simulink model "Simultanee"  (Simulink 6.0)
settings: Solver=ode45  StartTime=0  StopTime=3*t0  RelTol=1e-3
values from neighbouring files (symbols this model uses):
  beta = 0.95    [Constantes.m]    (also in ConstantesBck.m; ResCourV1.m = 1; ResCrV1.m = 1; ResEnerV1.m = 1)
  Cmem = 1E-6*Sm*(1-b)    (= 2.826e-08)    [Constantes.m]    (also in ConstantesBck.m = 3.14e-11; ImpedanceZtissus.m = 4e-08; Ztissus.m = 4e-08; CalculCharge.m = 1)
  N = [6,8,5,5,7,1,2,6,9,1,1,9,4,8,8,7]    [Constantes.m]    (also in ConstantesBck.m; ImpedanceZtissus.m = 100; Ztissus.m = 100; charge.m = N(:,2))
  rapportIE = 10    [Constantes.m]
  Rcan = 6.398E3*Sm*(1-b)    (= 180.80748)    [Constantes.m]    (also in ConstantesBck.m = 0.03454; ImpedanceZtissus.m = 44; Ztissus.m = 44)
  t0 = 2E-3    (= 0.002)    [Constantes.m]    (also in ConstantesBck.m = 0.001)
undefined symbols (not defined in the file or in its folder): ln
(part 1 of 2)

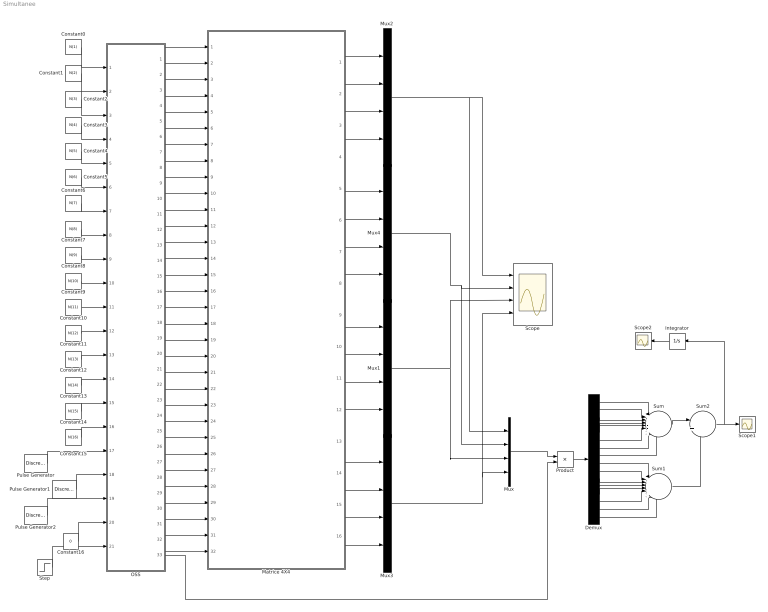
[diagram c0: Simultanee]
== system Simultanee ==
  Constant0 : Constant  Value=N(1)
  Constant1 : Constant  Value=N(2)
  Constant10 : Constant  Value=N(11)
  Constant11 : Constant  Value=N(12)
  Constant12 : Constant  Value=N(13)
  Constant13 : Constant  Value=N(14)
  Constant14 : Constant  Value=N(15)
  Constant15 : Constant  Value=N(16)
  Constant16 : Constant  Value=0
  Constant2 : Constant  Value=N(3)
  Constant3 : Constant  Value=N(4)
  Constant4 : Constant  Value=N(5)
  Constant5 : Constant  Value=N(6)
  Constant6 : Constant  Value=N(7)
  Constant7 : Constant  Value=N(8)
  Constant8 : Constant  Value=N(9)
  Constant9 : Constant  Value=N(10)
  Demux : Demux  Outputs=16
  Integrator : Integrator  Orientation=left
  Matrice 4X4 : Subsystem
  Mux{,1..4} (5 alike) : Mux
  OSS : Stateflow chart
  Product : Product
  Pulse Generator : DiscretePulseGenerator  PulseType=Time based  Period=2*t0  PulseWidth=50  PhaseDelay=2*t0
  Pulse Generator1 : DiscretePulseGenerator  PulseType=Time based  Period=4*t0  PulseWidth=50  PhaseDelay=3*t0
  Pulse Generator2 : DiscretePulseGenerator  PulseType=Time based  Period=8*t0  PulseWidth=50  PhaseDelay=5*t0
  Scope : Scope  NumInputPorts=4
  Scope1 : Scope
  Scope2 : Scope
  Step : Step  Time=t0  SampleTime=0
  Sum : Sum  Inputs=|++++++++
  Sum1 : Sum  Inputs=|++++++++
  Sum2 : Sum  Inputs=|++
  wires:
  Matrice 4X4/13(Out12) -> Mux3/1
  Matrice 4X4/14(Out13) -> Mux3/2
  Matrice 4X4/15(Out14) -> Mux3/3
  Matrice 4X4/16(Out15) -> Mux3/4
  Constant14/1 -> OSS/15(u14)
  Constant13/1 -> OSS/14(u13)
  Constant12/1 -> OSS/13(u12)
  Constant11/1 -> OSS/12(u11)
  Constant10/1 -> OSS/11(u10)
  Constant9/1 -> OSS/10(u9)
  Constant8/1 -> OSS/9(u8)
  Constant7/1 -> OSS/8(u7)
  Constant6/1 -> OSS/7(u6)
  Constant5/1 -> OSS/6(u5)
  Constant4/1 -> OSS/5(u4)
  Constant3/1 -> OSS/4(u3)
  Constant2/1 -> OSS/3(u2)
  Constant1/1 -> OSS/2(u1)
  Constant0/1 -> OSS/1(u0)
  Constant15/1 -> OSS/16(u15)
  OSS/5(S2) -> Matrice 4X4/5(S2)
  OSS/6(Ref2) -> Matrice 4X4/6(Ref2)
  OSS/7(S3) -> Matrice 4X4/7(S3)
  OSS/8(Ref3) -> Matrice 4X4/8(Ref3)
  OSS/9(S4) -> Matrice 4X4/9(S4)
  OSS/10(Ref4) -> Matrice 4X4/10(Ref4)
  OSS/11(S5) -> Matrice 4X4/11(S5)
  OSS/12(Ref5) -> Matrice 4X4/12(Ref5)
  OSS/13(S6) -> Matrice 4X4/13(S6)
  OSS/14(Ref6) -> Matrice 4X4/14(Ref6)
  OSS/15(S7) -> Matrice 4X4/15(S7)
  OSS/16(Ref7) -> Matrice 4X4/16(Ref7)
  OSS/17(S8) -> Matrice 4X4/17(S8)
  OSS/18(Ref8) -> Matrice 4X4/18(Ref8)
  OSS/19(S9) -> Matrice 4X4/19(S9)
  OSS/20(Ref9) -> Matrice 4X4/20(Ref9)
  OSS/21(S10) -> Matrice 4X4/21(S10)
  OSS/22(Ref10) -> Matrice 4X4/22(Ref10)
  OSS/23(S11) -> Matrice 4X4/23(S11)
  OSS/24(Ref11) -> Matrice 4X4/24(Ref11)
  OSS/25(S12) -> Matrice 4X4/25(S12)
  OSS/26(Ref12) -> Matrice 4X4/26(Ref12)
  OSS/27(S13) -> Matrice 4X4/27(S13)
  OSS/28(Ref13) -> Matrice 4X4/28(Ref13)
  OSS/29(S14) -> Matrice 4X4/29(S14)
  OSS/30(Ref14) -> Matrice 4X4/30(Ref14)
  OSS/31(S15) -> Matrice 4X4/31(S15)
  OSS/32(Ref15) -> Matrice 4X4/32(Ref15)
  OSS/4(Ref1) -> Matrice 4X4/4(Ref1)
  OSS/3(S1) -> Matrice 4X4/3(S1)
  OSS/2(Ref0) -> Matrice 4X4/2(Ref0)
  OSS/1(S0) -> Matrice 4X4/1(S0)
  Pulse Generator/1 -> OSS/17(tc0)
  Pulse Generator2/1 -> OSS/19(tc2)
  Pulse Generator1/1 -> OSS/18(tc1)
  Mux3/1 -> Mux/4, Scope/4
  Matrice 4X4/9(Out8) -> Mux1/1
  Matrice 4X4/10(Out9) -> Mux1/2
  Matrice 4X4/12(Out11) -> Mux1/4
  Matrice 4X4/11(Out10) -> Mux1/3
  Matrice 4X4/5(Out4) -> Mux4/1
  Matrice 4X4/6(Out5) -> Mux4/2
  Matrice 4X4/7(Out6) -> Mux4/3
  Matrice 4X4/8(Out7) -> Mux4/4
  Matrice 4X4/1(Out0) -> Mux2/1
  Matrice 4X4/2(Out1) -> Mux2/2
  Matrice 4X4/4(Out3) -> Mux2/4
  Matrice 4X4/3(Out2) -> Mux2/3
  Mux1/1 -> Mux/3, Scope/3
  Mux4/1 -> Mux/2, Scope/2
  Mux2/1 -> Mux/1, Scope/1
  Constant16/1 -> OSS/20(dyn)
  OSS/33(MatCourant) -> Product/2
  Mux/1 -> Product/1
  Product/1 -> Demux/1
  Demux/1 -> Sum/1
  Demux/2 -> Sum/2
  Demux/3 -> Sum/3
  Demux/4 -> Sum/4
  Demux/5 -> Sum/5
  Demux/6 -> Sum/6
  Demux/7 -> Sum/7
  Demux/8 -> Sum/8
  Demux/9 -> Sum1/1
  Demux/10 -> Sum1/2
  Demux/11 -> Sum1/3
  Demux/12 -> Sum1/4
  Demux/13 -> Sum1/5
  Demux/14 -> Sum1/6
  Demux/15 -> Sum1/7
  Demux/16 -> Sum1/8
  Sum/1 -> Sum2/1
  Sum1/1 -> Sum2/2
  Sum2/1 -> Scope1/1, Integrator/1
  Step/1 -> OSS/21(rst)
  Integrator/1 -> Scope2/1

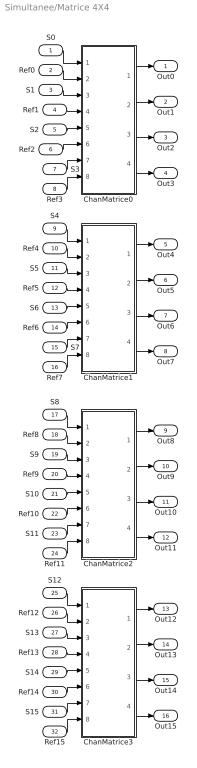
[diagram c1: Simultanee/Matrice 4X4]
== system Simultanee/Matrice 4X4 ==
  S0 : Inport  Port=1  LatchInput=off
  Ref0 : Inport  Port=2  LatchInput=off
  S1 : Inport  Port=3  LatchInput=off
  Ref1 : Inport  Port=4  LatchInput=off
  S2 : Inport  Port=5  LatchInput=off
  Ref2 : Inport  Port=6  LatchInput=off
  S3 : Inport  Port=7  LatchInput=off
  Ref3 : Inport  Port=8  LatchInput=off
  S4 : Inport  Port=9  LatchInput=off
  Ref4 : Inport  Port=10  LatchInput=off
  S5 : Inport  Port=11  LatchInput=off
  Ref5 : Inport  Port=12  LatchInput=off
  S6 : Inport  Port=13  LatchInput=off
  Ref6 : Inport  Port=14  LatchInput=off
  S7 : Inport  Port=15  LatchInput=off
  Ref7 : Inport  Port=16  LatchInput=off
  S8 : Inport  Port=17  LatchInput=off
  Ref8 : Inport  Port=18  LatchInput=off
  S9 : Inport  Port=19  LatchInput=off
  Ref9 : Inport  Port=20  LatchInput=off
  S10 : Inport  Port=21  LatchInput=off
  Ref10 : Inport  Port=22  LatchInput=off
  S11 : Inport  Port=23  LatchInput=off
  Ref11 : Inport  Port=24  LatchInput=off
  S12 : Inport  Port=25  LatchInput=off
  Ref12 : Inport  Port=26  LatchInput=off
  S13 : Inport  Port=27  LatchInput=off
  Ref13 : Inport  Port=28  LatchInput=off
  S14 : Inport  Port=29  LatchInput=off
  Ref14 : Inport  Port=30  LatchInput=off
  S15 : Inport  Port=31  LatchInput=off
  Ref15 : Inport  Port=32  LatchInput=off
  ChanMatrice0 : Subsystem
  ChanMatrice1 : Subsystem
  ChanMatrice2 : Subsystem
  ChanMatrice3 : Subsystem
  Out0 : Outport
  Out1 : Outport  Port=2
  Out2 : Outport  Port=3
  Out3 : Outport  Port=4
  Out4 : Outport  Port=5
  Out5 : Outport  Port=6
  Out6 : Outport  Port=7
  Out7 : Outport  Port=8
  Out8 : Outport  Port=9
  Out9 : Outport  Port=10
  Out10 : Outport  Port=11
  Out11 : Outport  Port=12
  Out12 : Outport  Port=13
  Out13 : Outport  Port=14
  Out14 : Outport  Port=15
  Out15 : Outport  Port=16
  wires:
  S0/1 -> ChanMatrice0/1(S0)
  ChanMatrice0/1(Out0) -> Out0/1
  Ref0/1 -> ChanMatrice0/2(Ref0)
  S1/1 -> ChanMatrice0/3(S1)
  ChanMatrice0/2(Out1) -> Out1/1
  ChanMatrice0/3(Out2) -> Out2/1
  ChanMatrice0/4(Out3) -> Out3/1
  ChanMatrice1/1(Out0) -> Out4/1
  ChanMatrice1/2(Out1) -> Out5/1
  ChanMatrice1/3(Out2) -> Out6/1
  ChanMatrice1/4(Out3) -> Out7/1
  ChanMatrice2/1(Out0) -> Out8/1
  ChanMatrice2/2(Out1) -> Out9/1
  ChanMatrice2/3(Out2) -> Out10/1
  ChanMatrice2/4(Out3) -> Out11/1
  ChanMatrice3/1(Out0) -> Out12/1
  ChanMatrice3/2(Out1) -> Out13/1
  ChanMatrice3/3(Out2) -> Out14/1
  ChanMatrice3/4(Out3) -> Out15/1
  S2/1 -> ChanMatrice0/5(S2)
  S3/1 -> ChanMatrice0/7(S3)
  S4/1 -> ChanMatrice1/1(S0)
  S5/1 -> ChanMatrice1/3(S1)
  S6/1 -> ChanMatrice1/5(S2)
  S7/1 -> ChanMatrice1/7(S3)
  S12/1 -> ChanMatrice3/1(S0)
  S13/1 -> ChanMatrice3/3(S1)
  S14/1 -> ChanMatrice3/5(S2)
  S15/1 -> ChanMatrice3/7(S3)
  S8/1 -> ChanMatrice2/1(S0)
  S9/1 -> ChanMatrice2/3(S1)
  S10/1 -> ChanMatrice2/5(S2)
  S11/1 -> ChanMatrice2/7(S3)
  Ref1/1 -> ChanMatrice0/4(Ref1)
  Ref2/1 -> ChanMatrice0/6(Ref2)
  Ref3/1 -> ChanMatrice0/8(Ref3)
  Ref4/1 -> ChanMatrice1/2(Ref0)
  Ref5/1 -> ChanMatrice1/4(Ref1)
  Ref6/1 -> ChanMatrice1/6(Ref2)
  Ref7/1 -> ChanMatrice1/8(Ref3)
  Ref8/1 -> ChanMatrice2/2(Ref0)
  Ref9/1 -> ChanMatrice2/4(Ref1)
  Ref10/1 -> ChanMatrice2/6(Ref2)
  Ref11/1 -> ChanMatrice2/8(Ref3)
  Ref12/1 -> ChanMatrice3/2(Ref0)
  Ref13/1 -> ChanMatrice3/4(Ref1)
  Ref14/1 -> ChanMatrice3/6(Ref2)
  Ref15/1 -> ChanMatrice3/8(Ref3)

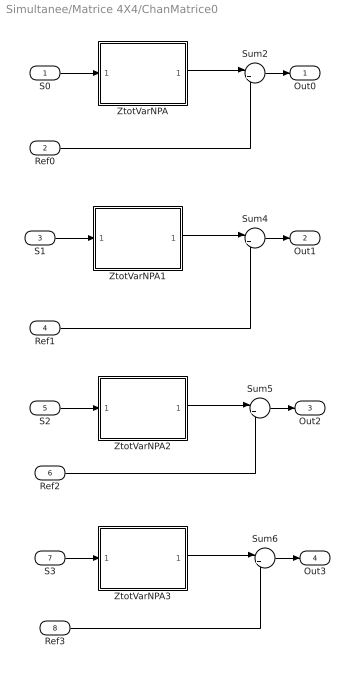
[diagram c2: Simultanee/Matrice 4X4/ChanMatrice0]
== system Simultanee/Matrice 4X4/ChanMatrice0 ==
  S0 : Inport  Port=1  LatchInput=off
  Ref0 : Inport  Port=2  LatchInput=off
  S1 : Inport  Port=3  LatchInput=off
  Ref1 : Inport  Port=4  LatchInput=off
  S2 : Inport  Port=5  LatchInput=off
  Ref2 : Inport  Port=6  LatchInput=off
  S3 : Inport  Port=7  LatchInput=off
  Ref3 : Inport  Port=8  LatchInput=off
  Sum{2,4..6} (4 alike) : Sum  Inputs=|++
  ZtotVarNPA : Subsystem
  ZtotVarNPA1 : Subsystem
  ZtotVarNPA2 : Subsystem
  ZtotVarNPA3 : Subsystem
  Out0 : Outport
  Out1 : Outport  Port=2
  Out2 : Outport  Port=3
  Out3 : Outport  Port=4
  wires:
  ZtotVarNPA/1(OutZtot) -> Sum2/1
  ZtotVarNPA1/1(OutZtot) -> Sum4/1
  ZtotVarNPA2/1(OutZtot) -> Sum5/1
  ZtotVarNPA3/1(OutZtot) -> Sum6/1
  Sum2/1 -> Out0/1
  S0/1 -> ZtotVarNPA/1(InZtot)
  Ref0/1 -> Sum2/2
  Sum4/1 -> Out1/1
  S1/1 -> ZtotVarNPA1/1(InZtot)
  Ref1/1 -> Sum4/2
  Sum5/1 -> Out2/1
  S2/1 -> ZtotVarNPA2/1(InZtot)
  Ref2/1 -> Sum5/2
  Sum6/1 -> Out3/1
  S3/1 -> ZtotVarNPA3/1(InZtot)
  Ref3/1 -> Sum6/2

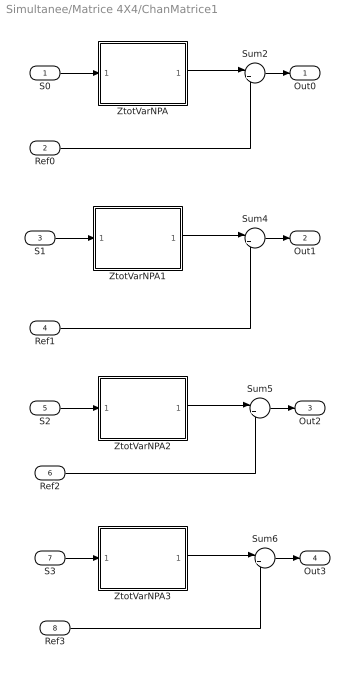
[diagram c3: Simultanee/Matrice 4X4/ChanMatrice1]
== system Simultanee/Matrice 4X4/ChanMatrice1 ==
  S0 : Inport  Port=1  LatchInput=off
  Ref0 : Inport  Port=2  LatchInput=off
  S1 : Inport  Port=3  LatchInput=off
  Ref1 : Inport  Port=4  LatchInput=off
  S2 : Inport  Port=5  LatchInput=off
  Ref2 : Inport  Port=6  LatchInput=off
  S3 : Inport  Port=7  LatchInput=off
  Ref3 : Inport  Port=8  LatchInput=off
  Sum{2,4..6} (4 alike) : Sum  Inputs=|++
  ZtotVarNPA : Subsystem
  ZtotVarNPA1 : Subsystem
  ZtotVarNPA2 : Subsystem
  ZtotVarNPA3 : Subsystem
  Out0 : Outport
  Out1 : Outport  Port=2
  Out2 : Outport  Port=3
  Out3 : Outport  Port=4
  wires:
  ZtotVarNPA/1(OutZtot) -> Sum2/1
  ZtotVarNPA1/1(OutZtot) -> Sum4/1
  ZtotVarNPA2/1(OutZtot) -> Sum5/1
  ZtotVarNPA3/1(OutZtot) -> Sum6/1
  Sum2/1 -> Out0/1
  S0/1 -> ZtotVarNPA/1(InZtot)
  Ref0/1 -> Sum2/2
  Sum4/1 -> Out1/1
  S1/1 -> ZtotVarNPA1/1(InZtot)
  Ref1/1 -> Sum4/2
  Sum5/1 -> Out2/1
  S2/1 -> ZtotVarNPA2/1(InZtot)
  Ref2/1 -> Sum5/2
  Sum6/1 -> Out3/1
  S3/1 -> ZtotVarNPA3/1(InZtot)
  Ref3/1 -> Sum6/2

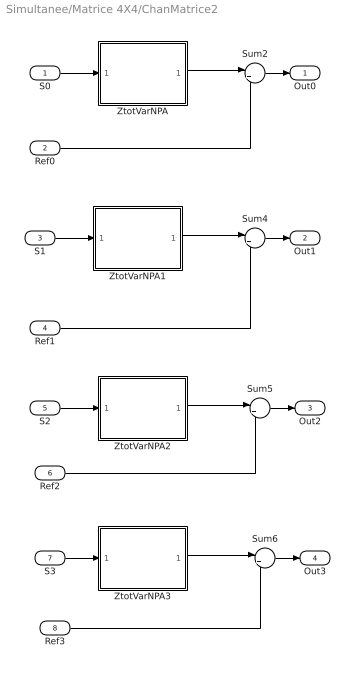
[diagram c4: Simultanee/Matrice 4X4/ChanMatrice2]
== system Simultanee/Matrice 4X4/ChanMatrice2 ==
  S0 : Inport  Port=1  LatchInput=off
  Ref0 : Inport  Port=2  LatchInput=off
  S1 : Inport  Port=3  LatchInput=off
  Ref1 : Inport  Port=4  LatchInput=off
  S2 : Inport  Port=5  LatchInput=off
  Ref2 : Inport  Port=6  LatchInput=off
  S3 : Inport  Port=7  LatchInput=off
  Ref3 : Inport  Port=8  LatchInput=off
  Sum{2,4..6} (4 alike) : Sum  Inputs=|++
  ZtotVarNPA : Subsystem
  ZtotVarNPA1 : Subsystem
  ZtotVarNPA2 : Subsystem
  ZtotVarNPA3 : Subsystem
  Out0 : Outport
  Out1 : Outport  Port=2
  Out2 : Outport  Port=3
  Out3 : Outport  Port=4
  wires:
  ZtotVarNPA/1(OutZtot) -> Sum2/1
  ZtotVarNPA1/1(OutZtot) -> Sum4/1
  ZtotVarNPA2/1(OutZtot) -> Sum5/1
  ZtotVarNPA3/1(OutZtot) -> Sum6/1
  Sum2/1 -> Out0/1
  S0/1 -> ZtotVarNPA/1(InZtot)
  Ref0/1 -> Sum2/2
  Sum4/1 -> Out1/1
  S1/1 -> ZtotVarNPA1/1(InZtot)
  Ref1/1 -> Sum4/2
  Sum5/1 -> Out2/1
  S2/1 -> ZtotVarNPA2/1(InZtot)
  Ref2/1 -> Sum5/2
  Sum6/1 -> Out3/1
  S3/1 -> ZtotVarNPA3/1(InZtot)
  Ref3/1 -> Sum6/2

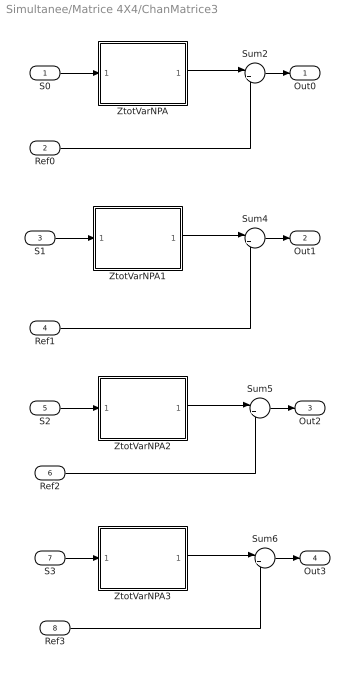
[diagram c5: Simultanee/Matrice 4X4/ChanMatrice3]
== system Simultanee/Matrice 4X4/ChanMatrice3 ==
  S0 : Inport  Port=1  LatchInput=off
  Ref0 : Inport  Port=2  LatchInput=off
  S1 : Inport  Port=3  LatchInput=off
  Ref1 : Inport  Port=4  LatchInput=off
  S2 : Inport  Port=5  LatchInput=off
  Ref2 : Inport  Port=6  LatchInput=off
  S3 : Inport  Port=7  LatchInput=off
  Ref3 : Inport  Port=8  LatchInput=off
  Sum{2,4..6} (4 alike) : Sum  Inputs=|++
  ZtotVarNPA : Subsystem
  ZtotVarNPA1 : Subsystem
  ZtotVarNPA2 : Subsystem
  ZtotVarNPA3 : Subsystem
  Out0 : Outport
  Out1 : Outport  Port=2
  Out2 : Outport  Port=3
  Out3 : Outport  Port=4
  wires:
  ZtotVarNPA/1(OutZtot) -> Sum2/1
  ZtotVarNPA1/1(OutZtot) -> Sum4/1
  ZtotVarNPA2/1(OutZtot) -> Sum5/1
  ZtotVarNPA3/1(OutZtot) -> Sum6/1
  Sum2/1 -> Out0/1
  S0/1 -> ZtotVarNPA/1(InZtot)
  Ref0/1 -> Sum2/2
  Sum4/1 -> Out1/1
  S1/1 -> ZtotVarNPA1/1(InZtot)
  Ref1/1 -> Sum4/2
  Sum5/1 -> Out2/1
  S2/1 -> ZtotVarNPA2/1(InZtot)
  Ref2/1 -> Sum5/2
  Sum6/1 -> Out3/1
  S3/1 -> ZtotVarNPA3/1(InZtot)
  Ref3/1 -> Sum6/2

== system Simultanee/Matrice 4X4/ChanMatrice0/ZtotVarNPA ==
  InZtot : Inport  Port=1  LatchInput=off
  Gain : Gain
  Sum : Sum  Inputs=|++
  ZietVar : Subsystem
  ZmembraneVar : Subsystem
  OutZtot : Outport
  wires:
  ZietVar/1(OutZiet) -> Gain/1
  ZmembraneVar/1(OutZmem) -> Sum/1
  InZtot/1 -> ZmembraneVar/1(InZmem), ZietVar/1(InZiet)
  Gain/1 -> Sum/2
  Sum/1 -> OutZtot/1

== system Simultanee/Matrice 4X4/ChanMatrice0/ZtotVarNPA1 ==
  InZtot : Inport  Port=1  LatchInput=off
  Gain : Gain
  Sum : Sum  Inputs=|++
  ZietVar : Subsystem
  ZmembraneVar : Subsystem
  OutZtot : Outport
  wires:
  ZietVar/1(OutZiet) -> Gain/1
  ZmembraneVar/1(OutZmem) -> Sum/1
  InZtot/1 -> ZmembraneVar/1(InZmem), ZietVar/1(InZiet)
  Gain/1 -> Sum/2
  Sum/1 -> OutZtot/1

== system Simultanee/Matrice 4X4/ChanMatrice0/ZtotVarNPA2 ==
  InZtot : Inport  Port=1  LatchInput=off
  Gain : Gain
  Sum : Sum  Inputs=|++
  ZietVar : Subsystem
  ZmembraneVar : Subsystem
  OutZtot : Outport
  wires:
  ZietVar/1(OutZiet) -> Gain/1
  ZmembraneVar/1(OutZmem) -> Sum/1
  InZtot/1 -> ZmembraneVar/1(InZmem), ZietVar/1(InZiet)
  Gain/1 -> Sum/2
  Sum/1 -> OutZtot/1

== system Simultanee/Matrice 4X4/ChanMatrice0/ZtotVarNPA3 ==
  InZtot : Inport  Port=1  LatchInput=off
  Gain : Gain
  Sum : Sum  Inputs=|++
  ZietVar : Subsystem
  ZmembraneVar : Subsystem
  OutZtot : Outport
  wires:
  ZietVar/1(OutZiet) -> Gain/1
  ZmembraneVar/1(OutZmem) -> Sum/1
  InZtot/1 -> ZmembraneVar/1(InZmem), ZietVar/1(InZiet)
  Gain/1 -> Sum/2
  Sum/1 -> OutZtot/1

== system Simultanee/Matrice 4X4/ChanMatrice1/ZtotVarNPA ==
  InZtot : Inport  Port=1  LatchInput=off
  Gain : Gain
  Sum : Sum  Inputs=|++
  ZietVar : Subsystem
  ZmembraneVar : Subsystem
  OutZtot : Outport
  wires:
  ZietVar/1(OutZiet) -> Gain/1
  ZmembraneVar/1(OutZmem) -> Sum/1
  InZtot/1 -> ZmembraneVar/1(InZmem), ZietVar/1(InZiet)
  Gain/1 -> Sum/2
  Sum/1 -> OutZtot/1

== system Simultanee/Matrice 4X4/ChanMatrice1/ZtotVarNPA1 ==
  InZtot : Inport  Port=1  LatchInput=off
  Gain : Gain
  Sum : Sum  Inputs=|++
  ZietVar : Subsystem
  ZmembraneVar : Subsystem
  OutZtot : Outport
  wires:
  ZietVar/1(OutZiet) -> Gain/1
  ZmembraneVar/1(OutZmem) -> Sum/1
  InZtot/1 -> ZmembraneVar/1(InZmem), ZietVar/1(InZiet)
  Gain/1 -> Sum/2
  Sum/1 -> OutZtot/1

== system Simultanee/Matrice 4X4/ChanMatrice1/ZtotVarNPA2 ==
  InZtot : Inport  Port=1  LatchInput=off
  Gain : Gain
  Sum : Sum  Inputs=|++
  ZietVar : Subsystem
  ZmembraneVar : Subsystem
  OutZtot : Outport
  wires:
  ZietVar/1(OutZiet) -> Gain/1
  ZmembraneVar/1(OutZmem) -> Sum/1
  InZtot/1 -> ZmembraneVar/1(InZmem), ZietVar/1(InZiet)
  Gain/1 -> Sum/2
  Sum/1 -> OutZtot/1

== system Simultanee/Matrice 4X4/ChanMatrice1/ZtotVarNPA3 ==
  InZtot : Inport  Port=1  LatchInput=off
  Gain : Gain
  Sum : Sum  Inputs=|++
  ZietVar : Subsystem
  ZmembraneVar : Subsystem
  OutZtot : Outport
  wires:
  ZietVar/1(OutZiet) -> Gain/1
  ZmembraneVar/1(OutZmem) -> Sum/1
  InZtot/1 -> ZmembraneVar/1(InZmem), ZietVar/1(InZiet)
  Gain/1 -> Sum/2
  Sum/1 -> OutZtot/1

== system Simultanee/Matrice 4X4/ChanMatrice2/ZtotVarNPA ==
  InZtot : Inport  Port=1  LatchInput=off
  Gain : Gain
  Sum : Sum  Inputs=|++
  ZietVar : Subsystem
  ZmembraneVar : Subsystem
  OutZtot : Outport
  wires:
  ZietVar/1(OutZiet) -> Gain/1
  ZmembraneVar/1(OutZmem) -> Sum/1
  InZtot/1 -> ZmembraneVar/1(InZmem), ZietVar/1(InZiet)
  Gain/1 -> Sum/2
  Sum/1 -> OutZtot/1

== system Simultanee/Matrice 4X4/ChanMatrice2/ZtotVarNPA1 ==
  InZtot : Inport  Port=1  LatchInput=off
  Gain : Gain
  Sum : Sum  Inputs=|++
  ZietVar : Subsystem
  ZmembraneVar : Subsystem
  OutZtot : Outport
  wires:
  ZietVar/1(OutZiet) -> Gain/1
  ZmembraneVar/1(OutZmem) -> Sum/1
  InZtot/1 -> ZmembraneVar/1(InZmem), ZietVar/1(InZiet)
  Gain/1 -> Sum/2
  Sum/1 -> OutZtot/1

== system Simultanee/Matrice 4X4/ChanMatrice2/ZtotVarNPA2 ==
  InZtot : Inport  Port=1  LatchInput=off
  Gain : Gain
  Sum : Sum  Inputs=|++
  ZietVar : Subsystem
  ZmembraneVar : Subsystem
  OutZtot : Outport
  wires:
  ZietVar/1(OutZiet) -> Gain/1
  ZmembraneVar/1(OutZmem) -> Sum/1
  InZtot/1 -> ZmembraneVar/1(InZmem), ZietVar/1(InZiet)
  Gain/1 -> Sum/2
  Sum/1 -> OutZtot/1

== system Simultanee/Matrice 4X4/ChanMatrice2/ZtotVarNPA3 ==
  InZtot : Inport  Port=1  LatchInput=off
  Gain : Gain
  Sum : Sum  Inputs=|++
  ZietVar : Subsystem
  ZmembraneVar : Subsystem
  OutZtot : Outport
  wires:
  ZietVar/1(OutZiet) -> Gain/1
  ZmembraneVar/1(OutZmem) -> Sum/1
  InZtot/1 -> ZmembraneVar/1(InZmem), ZietVar/1(InZiet)
  Gain/1 -> Sum/2
  Sum/1 -> OutZtot/1

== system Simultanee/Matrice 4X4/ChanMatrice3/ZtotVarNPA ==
  InZtot : Inport  Port=1  LatchInput=off
  Gain : Gain
  Sum : Sum  Inputs=|++
  ZietVar : Subsystem
  ZmembraneVar : Subsystem
  OutZtot : Outport
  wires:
  ZietVar/1(OutZiet) -> Gain/1
  ZmembraneVar/1(OutZmem) -> Sum/1
  InZtot/1 -> ZmembraneVar/1(InZmem), ZietVar/1(InZiet)
  Gain/1 -> Sum/2
  Sum/1 -> OutZtot/1

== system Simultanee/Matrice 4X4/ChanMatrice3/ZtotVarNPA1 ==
  InZtot : Inport  Port=1  LatchInput=off
  Gain : Gain
  Sum : Sum  Inputs=|++
  ZietVar : Subsystem
  ZmembraneVar : Subsystem
  OutZtot : Outport
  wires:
  ZietVar/1(OutZiet) -> Gain/1
  ZmembraneVar/1(OutZmem) -> Sum/1
  InZtot/1 -> ZmembraneVar/1(InZmem), ZietVar/1(InZiet)
  Gain/1 -> Sum/2
  Sum/1 -> OutZtot/1

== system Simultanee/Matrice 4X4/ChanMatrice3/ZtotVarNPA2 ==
  InZtot : Inport  Port=1  LatchInput=off
  Gain : Gain
  Sum : Sum  Inputs=|++
  ZietVar : Subsystem
  ZmembraneVar : Subsystem
  OutZtot : Outport
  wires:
  ZietVar/1(OutZiet) -> Gain/1
  ZmembraneVar/1(OutZmem) -> Sum/1
  InZtot/1 -> ZmembraneVar/1(InZmem), ZietVar/1(InZiet)
  Gain/1 -> Sum/2
  Sum/1 -> OutZtot/1

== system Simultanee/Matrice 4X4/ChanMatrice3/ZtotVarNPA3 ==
  InZtot : Inport  Port=1  LatchInput=off
  Gain : Gain
  Sum : Sum  Inputs=|++
  ZietVar : Subsystem
  ZmembraneVar : Subsystem
  OutZtot : Outport
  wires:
  ZietVar/1(OutZiet) -> Gain/1
  ZmembraneVar/1(OutZmem) -> Sum/1
  InZtot/1 -> ZmembraneVar/1(InZmem), ZietVar/1(InZiet)
  Gain/1 -> Sum/2
  Sum/1 -> OutZtot/1

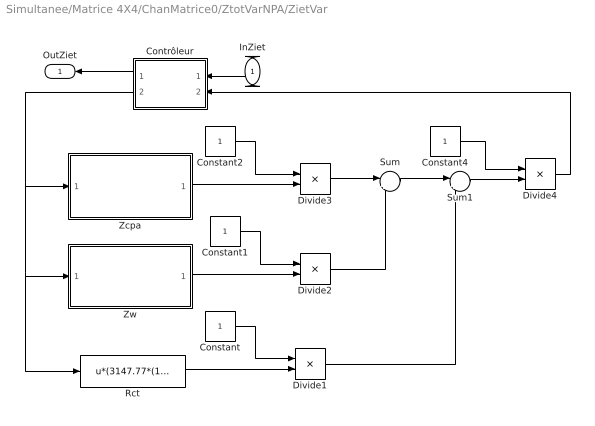
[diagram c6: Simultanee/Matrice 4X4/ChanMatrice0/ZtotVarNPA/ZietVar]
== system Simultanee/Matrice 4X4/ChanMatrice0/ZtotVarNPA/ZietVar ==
  InZiet : Inport  Orientation=left  Port=1  LatchInput=off
  Constant{,1..2,4} (4 alike) : Constant
  Contrôleur : Stateflow chart  Orientation=left
  Divide{1..4} (4 alike) : Product  Inputs=*/  OutScaling=2^-10
  Rct : Fcn  Expr=u*(3147.77*(1/((1E6*abs(u))^0.7199)))*1000
  Sum : Sum  Inputs=|++
  Sum1 : Sum  Inputs=|++
  Zcpa : Subsystem
  Zw : Subsystem
  OutZiet : Outport  Orientation=left
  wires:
  Constant/1 -> Divide1/1
  Constant1/1 -> Divide2/1
  Constant2/1 -> Divide3/1
  Zcpa/1(OutZcpa) -> Divide3/2
  Zw/1(OutZw) -> Divide2/2
  Rct/1 -> Divide1/2
  Divide3/1 -> Sum/1
  Constant4/1 -> Divide4/1
  Divide2/1 -> Sum/2
  Sum/1 -> Sum1/1
  Divide1/1 -> Sum1/2
  Sum1/1 -> Divide4/2
  Contrôleur/2(temp) -> Rct/1, Zw/1(InZw), Zcpa/1(InZcpa)
  InZiet/1 -> Contrôleur/1(u)
  Contrôleur/1(y) -> OutZiet/1
  Divide4/1 -> Contrôleur/2(calc)

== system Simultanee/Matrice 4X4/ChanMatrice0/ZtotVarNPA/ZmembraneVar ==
  InZmem : Inport  Orientation=left  Port=1  LatchInput=off
  Constant : Constant
  Constant1 : Constant
  Constant2 : Constant
  Contrôleur : Stateflow chart  Orientation=left
  Divide : Product  Inputs=*/  OutScaling=2^-10
  Divide1 : Product  Inputs=*/  OutScaling=2^-10
  Divide2 : Product  Inputs=*/  OutScaling=2^-10
  Gain : Gain  Gain=2
  Rext : Fcn  Expr=u*(1.6342*((abs(u)*1E6)^0.1267))*1E3
  Rint : Fcn  Expr=u*(1.6342*((abs(u)*1E6)^0.1267))*1E3/rapportIE
  Sum : Sum  Inputs=|++
  Sum1 : Sum  Inputs=|++
  Transfer Fcn : TransferFcn  Numerator=[Rcan]  Denominator=[Rcan*Cmem 1]
  OutZmem : Outport  Orientation=left
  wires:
  Gain/1 -> Transfer Fcn/1
  Transfer Fcn/1 -> Sum/1
  Sum/1 -> Divide/2
  Rext/1 -> Divide1/2
  Constant1/1 -> Divide/1
  Constant/1 -> Divide1/1
  Divide/1 -> Sum1/1
  Constant2/1 -> Divide2/1
  Sum1/1 -> Divide2/2
  Rint/1 -> Sum/2
  Divide1/1 -> Sum1/2
  Contrôleur/2(temp) -> Rext/1, Rint/1, Gain/1
  Divide2/1 -> Contrôleur/2(calc)
  InZmem/1 -> Contrôleur/1(u)
  Contrôleur/1(y) -> OutZmem/1

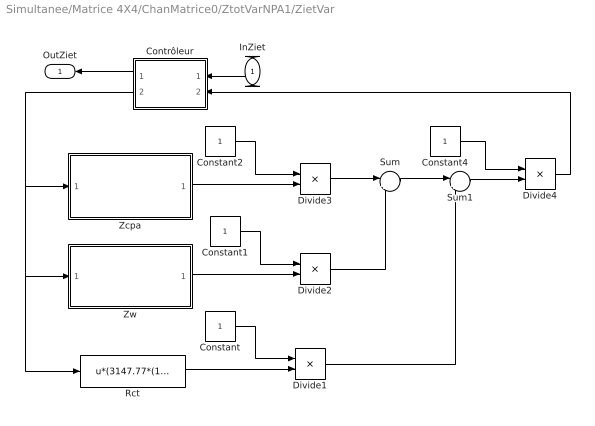
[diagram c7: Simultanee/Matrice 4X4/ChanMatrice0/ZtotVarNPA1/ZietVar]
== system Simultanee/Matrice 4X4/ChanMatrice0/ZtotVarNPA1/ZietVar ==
  InZiet : Inport  Orientation=left  Port=1  LatchInput=off
  Constant{,1..2,4} (4 alike) : Constant
  Contrôleur : Stateflow chart  Orientation=left
  Divide{1..4} (4 alike) : Product  Inputs=*/  OutScaling=2^-10
  Rct : Fcn  Expr=u*(3147.77*(1/((1E6*abs(u))^0.7199)))*1000
  Sum : Sum  Inputs=|++
  Sum1 : Sum  Inputs=|++
  Zcpa : Subsystem
  Zw : Subsystem
  OutZiet : Outport  Orientation=left
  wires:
  Constant/1 -> Divide1/1
  Constant1/1 -> Divide2/1
  Constant2/1 -> Divide3/1
  Zcpa/1(OutZcpa) -> Divide3/2
  Zw/1(OutZw) -> Divide2/2
  Rct/1 -> Divide1/2
  Divide3/1 -> Sum/1
  Constant4/1 -> Divide4/1
  Divide2/1 -> Sum/2
  Sum/1 -> Sum1/1
  Divide1/1 -> Sum1/2
  Sum1/1 -> Divide4/2
  Contrôleur/2(temp) -> Rct/1, Zw/1(InZw), Zcpa/1(InZcpa)
  InZiet/1 -> Contrôleur/1(u)
  Contrôleur/1(y) -> OutZiet/1
  Divide4/1 -> Contrôleur/2(calc)

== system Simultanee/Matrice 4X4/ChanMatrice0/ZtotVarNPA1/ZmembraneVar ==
  InZmem : Inport  Orientation=left  Port=1  LatchInput=off
  Constant : Constant
  Constant1 : Constant
  Constant2 : Constant
  Contrôleur : Stateflow chart  Orientation=left
  Divide : Product  Inputs=*/  OutScaling=2^-10
  Divide1 : Product  Inputs=*/  OutScaling=2^-10
  Divide2 : Product  Inputs=*/  OutScaling=2^-10
  Gain : Gain  Gain=2
  Rext : Fcn  Expr=u*(1.6342*((abs(u)*1E6)^0.1267))*1E3
  Rint : Fcn  Expr=u*(1.6342*((abs(u)*1E6)^0.1267))*1E3/rapportIE
  Sum : Sum  Inputs=|++
  Sum1 : Sum  Inputs=|++
  Transfer Fcn : TransferFcn  Numerator=[Rcan]  Denominator=[Rcan*Cmem 1]
  OutZmem : Outport  Orientation=left
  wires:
  Gain/1 -> Transfer Fcn/1
  Transfer Fcn/1 -> Sum/1
  Sum/1 -> Divide/2
  Rext/1 -> Divide1/2
  Constant1/1 -> Divide/1
  Constant/1 -> Divide1/1
  Divide/1 -> Sum1/1
  Constant2/1 -> Divide2/1
  Sum1/1 -> Divide2/2
  Rint/1 -> Sum/2
  Divide1/1 -> Sum1/2
  Contrôleur/2(temp) -> Rext/1, Rint/1, Gain/1
  Divide2/1 -> Contrôleur/2(calc)
  InZmem/1 -> Contrôleur/1(u)
  Contrôleur/1(y) -> OutZmem/1

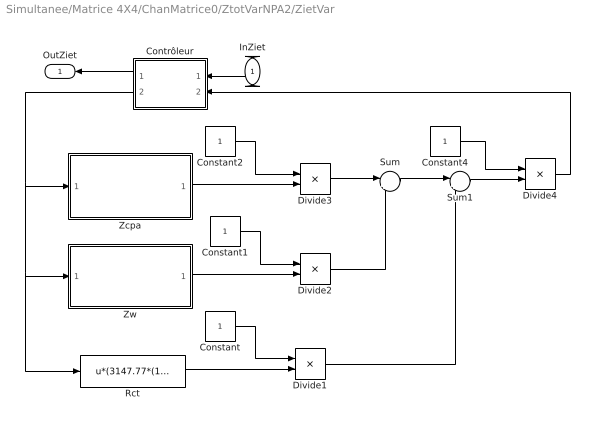
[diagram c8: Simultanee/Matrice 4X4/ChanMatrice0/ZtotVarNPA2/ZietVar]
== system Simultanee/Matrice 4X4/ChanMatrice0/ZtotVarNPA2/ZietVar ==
  InZiet : Inport  Orientation=left  Port=1  LatchInput=off
  Constant{,1..2,4} (4 alike) : Constant
  Contrôleur : Stateflow chart  Orientation=left
  Divide{1..4} (4 alike) : Product  Inputs=*/  OutScaling=2^-10
  Rct : Fcn  Expr=u*(3147.77*(1/((1E6*abs(u))^0.7199)))*1000
  Sum : Sum  Inputs=|++
  Sum1 : Sum  Inputs=|++
  Zcpa : Subsystem
  Zw : Subsystem
  OutZiet : Outport  Orientation=left
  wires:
  Constant/1 -> Divide1/1
  Constant1/1 -> Divide2/1
  Constant2/1 -> Divide3/1
  Zcpa/1(OutZcpa) -> Divide3/2
  Zw/1(OutZw) -> Divide2/2
  Rct/1 -> Divide1/2
  Divide3/1 -> Sum/1
  Constant4/1 -> Divide4/1
  Divide2/1 -> Sum/2
  Sum/1 -> Sum1/1
  Divide1/1 -> Sum1/2
  Sum1/1 -> Divide4/2
  Contrôleur/2(temp) -> Rct/1, Zw/1(InZw), Zcpa/1(InZcpa)
  InZiet/1 -> Contrôleur/1(u)
  Contrôleur/1(y) -> OutZiet/1
  Divide4/1 -> Contrôleur/2(calc)

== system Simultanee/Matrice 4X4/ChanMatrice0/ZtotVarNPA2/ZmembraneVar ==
  InZmem : Inport  Orientation=left  Port=1  LatchInput=off
  Constant : Constant
  Constant1 : Constant
  Constant2 : Constant
  Contrôleur : Stateflow chart  Orientation=left
  Divide : Product  Inputs=*/  OutScaling=2^-10
  Divide1 : Product  Inputs=*/  OutScaling=2^-10
  Divide2 : Product  Inputs=*/  OutScaling=2^-10
  Gain : Gain  Gain=2
  Rext : Fcn  Expr=u*(1.6342*((abs(u)*1E6)^0.1267))*1E3
  Rint : Fcn  Expr=u*(1.6342*((abs(u)*1E6)^0.1267))*1E3/rapportIE
  Sum : Sum  Inputs=|++
  Sum1 : Sum  Inputs=|++
  Transfer Fcn : TransferFcn  Numerator=[Rcan]  Denominator=[Rcan*Cmem 1]
  OutZmem : Outport  Orientation=left
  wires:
  Gain/1 -> Transfer Fcn/1
  Transfer Fcn/1 -> Sum/1
  Sum/1 -> Divide/2
  Rext/1 -> Divide1/2
  Constant1/1 -> Divide/1
  Constant/1 -> Divide1/1
  Divide/1 -> Sum1/1
  Constant2/1 -> Divide2/1
  Sum1/1 -> Divide2/2
  Rint/1 -> Sum/2
  Divide1/1 -> Sum1/2
  Contrôleur/2(temp) -> Rext/1, Rint/1, Gain/1
  Divide2/1 -> Contrôleur/2(calc)
  InZmem/1 -> Contrôleur/1(u)
  Contrôleur/1(y) -> OutZmem/1

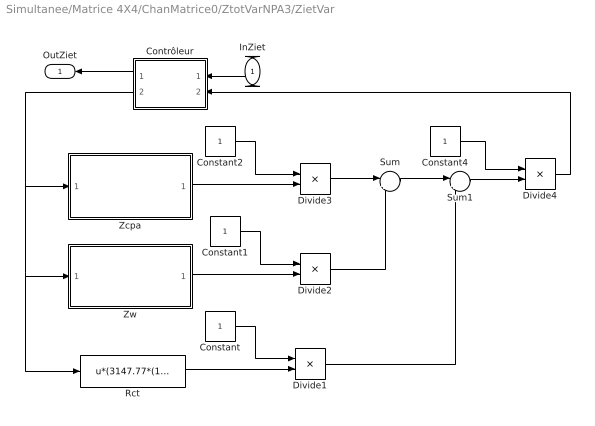
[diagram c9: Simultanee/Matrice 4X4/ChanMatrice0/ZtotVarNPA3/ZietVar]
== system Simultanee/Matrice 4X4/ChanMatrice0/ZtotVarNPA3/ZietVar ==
  InZiet : Inport  Orientation=left  Port=1  LatchInput=off
  Constant{,1..2,4} (4 alike) : Constant
  Contrôleur : Stateflow chart  Orientation=left
  Divide{1..4} (4 alike) : Product  Inputs=*/  OutScaling=2^-10
  Rct : Fcn  Expr=u*(3147.77*(1/((1E6*abs(u))^0.7199)))*1000
  Sum : Sum  Inputs=|++
  Sum1 : Sum  Inputs=|++
  Zcpa : Subsystem
  Zw : Subsystem
  OutZiet : Outport  Orientation=left
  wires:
  Constant/1 -> Divide1/1
  Constant1/1 -> Divide2/1
  Constant2/1 -> Divide3/1
  Zcpa/1(OutZcpa) -> Divide3/2
  Zw/1(OutZw) -> Divide2/2
  Rct/1 -> Divide1/2
  Divide3/1 -> Sum/1
  Constant4/1 -> Divide4/1
  Divide2/1 -> Sum/2
  Sum/1 -> Sum1/1
  Divide1/1 -> Sum1/2
  Sum1/1 -> Divide4/2
  Contrôleur/2(temp) -> Rct/1, Zw/1(InZw), Zcpa/1(InZcpa)
  InZiet/1 -> Contrôleur/1(u)
  Contrôleur/1(y) -> OutZiet/1
  Divide4/1 -> Contrôleur/2(calc)

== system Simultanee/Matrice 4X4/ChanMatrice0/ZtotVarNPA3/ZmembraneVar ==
  InZmem : Inport  Orientation=left  Port=1  LatchInput=off
  Constant : Constant
  Constant1 : Constant
  Constant2 : Constant
  Contrôleur : Stateflow chart  Orientation=left
  Divide : Product  Inputs=*/  OutScaling=2^-10
  Divide1 : Product  Inputs=*/  OutScaling=2^-10
  Divide2 : Product  Inputs=*/  OutScaling=2^-10
  Gain : Gain  Gain=2
  Rext : Fcn  Expr=u*(1.6342*((abs(u)*1E6)^0.1267))*1E3
  Rint : Fcn  Expr=u*(1.6342*((abs(u)*1E6)^0.1267))*1E3/rapportIE
  Sum : Sum  Inputs=|++
  Sum1 : Sum  Inputs=|++
  Transfer Fcn : TransferFcn  Numerator=[Rcan]  Denominator=[Rcan*Cmem 1]
  OutZmem : Outport  Orientation=left
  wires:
  Gain/1 -> Transfer Fcn/1
  Transfer Fcn/1 -> Sum/1
  Sum/1 -> Divide/2
  Rext/1 -> Divide1/2
  Constant1/1 -> Divide/1
  Constant/1 -> Divide1/1
  Divide/1 -> Sum1/1
  Constant2/1 -> Divide2/1
  Sum1/1 -> Divide2/2
  Rint/1 -> Sum/2
  Divide1/1 -> Sum1/2
  Contrôleur/2(temp) -> Rext/1, Rint/1, Gain/1
  Divide2/1 -> Contrôleur/2(calc)
  InZmem/1 -> Contrôleur/1(u)
  Contrôleur/1(y) -> OutZmem/1

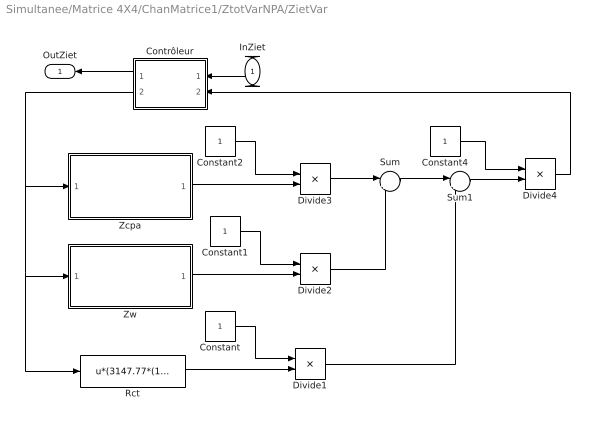
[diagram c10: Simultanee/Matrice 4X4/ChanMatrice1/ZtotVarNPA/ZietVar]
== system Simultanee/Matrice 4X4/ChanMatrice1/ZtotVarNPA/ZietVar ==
  InZiet : Inport  Orientation=left  Port=1  LatchInput=off
  Constant{,1..2,4} (4 alike) : Constant
  Contrôleur : Stateflow chart  Orientation=left
  Divide{1..4} (4 alike) : Product  Inputs=*/  OutScaling=2^-10
  Rct : Fcn  Expr=u*(3147.77*(1/((1E6*abs(u))^0.7199)))*1000
  Sum : Sum  Inputs=|++
  Sum1 : Sum  Inputs=|++
  Zcpa : Subsystem
  Zw : Subsystem
  OutZiet : Outport  Orientation=left
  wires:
  Constant/1 -> Divide1/1
  Constant1/1 -> Divide2/1
  Constant2/1 -> Divide3/1
  Zcpa/1(OutZcpa) -> Divide3/2
  Zw/1(OutZw) -> Divide2/2
  Rct/1 -> Divide1/2
  Divide3/1 -> Sum/1
  Constant4/1 -> Divide4/1
  Divide2/1 -> Sum/2
  Sum/1 -> Sum1/1
  Divide1/1 -> Sum1/2
  Sum1/1 -> Divide4/2
  Contrôleur/2(temp) -> Rct/1, Zw/1(InZw), Zcpa/1(InZcpa)
  InZiet/1 -> Contrôleur/1(u)
  Contrôleur/1(y) -> OutZiet/1
  Divide4/1 -> Contrôleur/2(calc)

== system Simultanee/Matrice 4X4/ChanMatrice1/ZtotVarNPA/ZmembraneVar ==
  InZmem : Inport  Orientation=left  Port=1  LatchInput=off
  Constant : Constant
  Constant1 : Constant
  Constant2 : Constant
  Contrôleur : Stateflow chart  Orientation=left
  Divide : Product  Inputs=*/  OutScaling=2^-10
  Divide1 : Product  Inputs=*/  OutScaling=2^-10
  Divide2 : Product  Inputs=*/  OutScaling=2^-10
  Gain : Gain  Gain=2
  Rext : Fcn  Expr=u*(1.6342*((abs(u)*1E6)^0.1267))*1E3
  Rint : Fcn  Expr=u*(1.6342*((abs(u)*1E6)^0.1267))*1E3/rapportIE
  Sum : Sum  Inputs=|++
  Sum1 : Sum  Inputs=|++
  Transfer Fcn : TransferFcn  Numerator=[Rcan]  Denominator=[Rcan*Cmem 1]
  OutZmem : Outport  Orientation=left
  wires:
  Gain/1 -> Transfer Fcn/1
  Transfer Fcn/1 -> Sum/1
  Sum/1 -> Divide/2
  Rext/1 -> Divide1/2
  Constant1/1 -> Divide/1
  Constant/1 -> Divide1/1
  Divide/1 -> Sum1/1
  Constant2/1 -> Divide2/1
  Sum1/1 -> Divide2/2
  Rint/1 -> Sum/2
  Divide1/1 -> Sum1/2
  Contrôleur/2(temp) -> Rext/1, Rint/1, Gain/1
  Divide2/1 -> Contrôleur/2(calc)
  InZmem/1 -> Contrôleur/1(u)
  Contrôleur/1(y) -> OutZmem/1

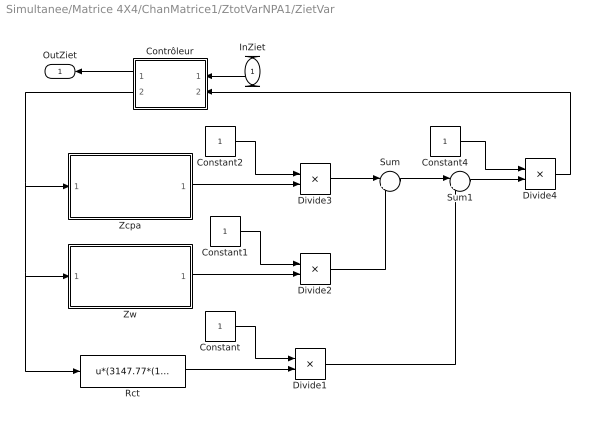
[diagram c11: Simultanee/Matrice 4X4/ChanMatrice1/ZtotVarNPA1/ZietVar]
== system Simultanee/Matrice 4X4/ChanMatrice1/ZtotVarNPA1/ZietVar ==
  InZiet : Inport  Orientation=left  Port=1  LatchInput=off
  Constant{,1..2,4} (4 alike) : Constant
  Contrôleur : Stateflow chart  Orientation=left
  Divide{1..4} (4 alike) : Product  Inputs=*/  OutScaling=2^-10
  Rct : Fcn  Expr=u*(3147.77*(1/((1E6*abs(u))^0.7199)))*1000
  Sum : Sum  Inputs=|++
  Sum1 : Sum  Inputs=|++
  Zcpa : Subsystem
  Zw : Subsystem
  OutZiet : Outport  Orientation=left
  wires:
  Constant/1 -> Divide1/1
  Constant1/1 -> Divide2/1
  Constant2/1 -> Divide3/1
  Zcpa/1(OutZcpa) -> Divide3/2
  Zw/1(OutZw) -> Divide2/2
  Rct/1 -> Divide1/2
  Divide3/1 -> Sum/1
  Constant4/1 -> Divide4/1
  Divide2/1 -> Sum/2
  Sum/1 -> Sum1/1
  Divide1/1 -> Sum1/2
  Sum1/1 -> Divide4/2
  Contrôleur/2(temp) -> Rct/1, Zw/1(InZw), Zcpa/1(InZcpa)
  InZiet/1 -> Contrôleur/1(u)
  Contrôleur/1(y) -> OutZiet/1
  Divide4/1 -> Contrôleur/2(calc)

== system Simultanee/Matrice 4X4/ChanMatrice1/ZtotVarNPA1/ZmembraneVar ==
  InZmem : Inport  Orientation=left  Port=1  LatchInput=off
  Constant : Constant
  Constant1 : Constant
  Constant2 : Constant
  Contrôleur : Stateflow chart  Orientation=left
  Divide : Product  Inputs=*/  OutScaling=2^-10
  Divide1 : Product  Inputs=*/  OutScaling=2^-10
  Divide2 : Product  Inputs=*/  OutScaling=2^-10
  Gain : Gain  Gain=2
  Rext : Fcn  Expr=u*(1.6342*((abs(u)*1E6)^0.1267))*1E3
  Rint : Fcn  Expr=u*(1.6342*((abs(u)*1E6)^0.1267))*1E3/rapportIE
  Sum : Sum  Inputs=|++
  Sum1 : Sum  Inputs=|++
  Transfer Fcn : TransferFcn  Numerator=[Rcan]  Denominator=[Rcan*Cmem 1]
  OutZmem : Outport  Orientation=left
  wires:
  Gain/1 -> Transfer Fcn/1
  Transfer Fcn/1 -> Sum/1
  Sum/1 -> Divide/2
  Rext/1 -> Divide1/2
  Constant1/1 -> Divide/1
  Constant/1 -> Divide1/1
  Divide/1 -> Sum1/1
  Constant2/1 -> Divide2/1
  Sum1/1 -> Divide2/2
  Rint/1 -> Sum/2
  Divide1/1 -> Sum1/2
  Contrôleur/2(temp) -> Rext/1, Rint/1, Gain/1
  Divide2/1 -> Contrôleur/2(calc)
  InZmem/1 -> Contrôleur/1(u)
  Contrôleur/1(y) -> OutZmem/1

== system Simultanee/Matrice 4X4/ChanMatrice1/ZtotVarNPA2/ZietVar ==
  InZiet : Inport  Orientation=left  Port=1  LatchInput=off
  Constant{,1..2,4} (4 alike) : Constant
  Contrôleur : Stateflow chart  Orientation=left
  Divide{1..4} (4 alike) : Product  Inputs=*/  OutScaling=2^-10
  Rct : Fcn  Expr=u*(3147.77*(1/((1E6*abs(u))^0.7199)))*1000
  Sum : Sum  Inputs=|++
  Sum1 : Sum  Inputs=|++
  Zcpa : Subsystem
  Zw : Subsystem
  OutZiet : Outport  Orientation=left
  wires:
  Constant/1 -> Divide1/1
  Constant1/1 -> Divide2/1
  Constant2/1 -> Divide3/1
  Zcpa/1(OutZcpa) -> Divide3/2
  Zw/1(OutZw) -> Divide2/2
  Rct/1 -> Divide1/2
  Divide3/1 -> Sum/1
  Constant4/1 -> Divide4/1
  Divide2/1 -> Sum/2
  Sum/1 -> Sum1/1
  Divide1/1 -> Sum1/2
  Sum1/1 -> Divide4/2
  Contrôleur/2(temp) -> Rct/1, Zw/1(InZw), Zcpa/1(InZcpa)
  InZiet/1 -> Contrôleur/1(u)
  Contrôleur/1(y) -> OutZiet/1
  Divide4/1 -> Contrôleur/2(calc)

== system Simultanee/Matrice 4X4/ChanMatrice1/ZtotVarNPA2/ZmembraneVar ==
  InZmem : Inport  Orientation=left  Port=1  LatchInput=off
  Constant : Constant
  Constant1 : Constant
  Constant2 : Constant
  Contrôleur : Stateflow chart  Orientation=left
  Divide : Product  Inputs=*/  OutScaling=2^-10
  Divide1 : Product  Inputs=*/  OutScaling=2^-10
  Divide2 : Product  Inputs=*/  OutScaling=2^-10
  Gain : Gain  Gain=2
  Rext : Fcn  Expr=u*(1.6342*((abs(u)*1E6)^0.1267))*1E3
  Rint : Fcn  Expr=u*(1.6342*((abs(u)*1E6)^0.1267))*1E3/rapportIE
  Sum : Sum  Inputs=|++
  Sum1 : Sum  Inputs=|++
  Transfer Fcn : TransferFcn  Numerator=[Rcan]  Denominator=[Rcan*Cmem 1]
  OutZmem : Outport  Orientation=left
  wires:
  Gain/1 -> Transfer Fcn/1
  Transfer Fcn/1 -> Sum/1
  Sum/1 -> Divide/2
  Rext/1 -> Divide1/2
  Constant1/1 -> Divide/1
  Constant/1 -> Divide1/1
  Divide/1 -> Sum1/1
  Constant2/1 -> Divide2/1
  Sum1/1 -> Divide2/2
  Rint/1 -> Sum/2
  Divide1/1 -> Sum1/2
  Contrôleur/2(temp) -> Rext/1, Rint/1, Gain/1
  Divide2/1 -> Contrôleur/2(calc)
  InZmem/1 -> Contrôleur/1(u)
  Contrôleur/1(y) -> OutZmem/1

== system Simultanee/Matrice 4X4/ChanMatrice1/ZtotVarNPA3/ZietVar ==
  InZiet : Inport  Orientation=left  Port=1  LatchInput=off
  Constant{,1..2,4} (4 alike) : Constant
  Contrôleur : Stateflow chart  Orientation=left
  Divide{1..4} (4 alike) : Product  Inputs=*/  OutScaling=2^-10
  Rct : Fcn  Expr=u*(3147.77*(1/((1E6*abs(u))^0.7199)))*1000
  Sum : Sum  Inputs=|++
  Sum1 : Sum  Inputs=|++
  Zcpa : Subsystem
  Zw : Subsystem
  OutZiet : Outport  Orientation=left
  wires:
  Constant/1 -> Divide1/1
  Constant1/1 -> Divide2/1
  Constant2/1 -> Divide3/1
  Zcpa/1(OutZcpa) -> Divide3/2
  Zw/1(OutZw) -> Divide2/2
  Rct/1 -> Divide1/2
  Divide3/1 -> Sum/1
  Constant4/1 -> Divide4/1
  Divide2/1 -> Sum/2
  Sum/1 -> Sum1/1
  Divide1/1 -> Sum1/2
  Sum1/1 -> Divide4/2
  Contrôleur/2(temp) -> Rct/1, Zw/1(InZw), Zcpa/1(InZcpa)
  InZiet/1 -> Contrôleur/1(u)
  Contrôleur/1(y) -> OutZiet/1
  Divide4/1 -> Contrôleur/2(calc)

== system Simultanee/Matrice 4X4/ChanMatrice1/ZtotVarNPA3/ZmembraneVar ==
  InZmem : Inport  Orientation=left  Port=1  LatchInput=off
  Constant : Constant
  Constant1 : Constant
  Constant2 : Constant
  Contrôleur : Stateflow chart  Orientation=left
  Divide : Product  Inputs=*/  OutScaling=2^-10
  Divide1 : Product  Inputs=*/  OutScaling=2^-10
  Divide2 : Product  Inputs=*/  OutScaling=2^-10
  Gain : Gain  Gain=2
  Rext : Fcn  Expr=u*(1.6342*((abs(u)*1E6)^0.1267))*1E3
  Rint : Fcn  Expr=u*(1.6342*((abs(u)*1E6)^0.1267))*1E3/rapportIE
  Sum : Sum  Inputs=|++
  Sum1 : Sum  Inputs=|++
  Transfer Fcn : TransferFcn  Numerator=[Rcan]  Denominator=[Rcan*Cmem 1]
  OutZmem : Outport  Orientation=left
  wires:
  Gain/1 -> Transfer Fcn/1
  Transfer Fcn/1 -> Sum/1
  Sum/1 -> Divide/2
  Rext/1 -> Divide1/2
  Constant1/1 -> Divide/1
  Constant/1 -> Divide1/1
  Divide/1 -> Sum1/1
  Constant2/1 -> Divide2/1
  Sum1/1 -> Divide2/2
  Rint/1 -> Sum/2
  Divide1/1 -> Sum1/2
  Contrôleur/2(temp) -> Rext/1, Rint/1, Gain/1
  Divide2/1 -> Contrôleur/2(calc)
  InZmem/1 -> Contrôleur/1(u)
  Contrôleur/1(y) -> OutZmem/1

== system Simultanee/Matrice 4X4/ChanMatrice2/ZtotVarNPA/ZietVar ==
  InZiet : Inport  Orientation=left  Port=1  LatchInput=off
  Constant{,1..2,4} (4 alike) : Constant
  Contrôleur : Stateflow chart  Orientation=left
  Divide{1..4} (4 alike) : Product  Inputs=*/  OutScaling=2^-10
  Rct : Fcn  Expr=u*(3147.77*(1/((1E6*abs(u))^0.7199)))*1000
  Sum : Sum  Inputs=|++
  Sum1 : Sum  Inputs=|++
  Zcpa : Subsystem
  Zw : Subsystem
  OutZiet : Outport  Orientation=left
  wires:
  Constant/1 -> Divide1/1
  Constant1/1 -> Divide2/1
  Constant2/1 -> Divide3/1
  Zcpa/1(OutZcpa) -> Divide3/2
  Zw/1(OutZw) -> Divide2/2
  Rct/1 -> Divide1/2
  Divide3/1 -> Sum/1
  Constant4/1 -> Divide4/1
  Divide2/1 -> Sum/2
  Sum/1 -> Sum1/1
  Divide1/1 -> Sum1/2
  Sum1/1 -> Divide4/2
  Contrôleur/2(temp) -> Rct/1, Zw/1(InZw), Zcpa/1(InZcpa)
  InZiet/1 -> Contrôleur/1(u)
  Contrôleur/1(y) -> OutZiet/1
  Divide4/1 -> Contrôleur/2(calc)

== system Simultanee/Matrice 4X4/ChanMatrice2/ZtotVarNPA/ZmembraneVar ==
  InZmem : Inport  Orientation=left  Port=1  LatchInput=off
  Constant : Constant
  Constant1 : Constant
  Constant2 : Constant
  Contrôleur : Stateflow chart  Orientation=left
  Divide : Product  Inputs=*/  OutScaling=2^-10
  Divide1 : Product  Inputs=*/  OutScaling=2^-10
  Divide2 : Product  Inputs=*/  OutScaling=2^-10
  Gain : Gain  Gain=2
  Rext : Fcn  Expr=u*(1.6342*((abs(u)*1E6)^0.1267))*1E3
  Rint : Fcn  Expr=u*(1.6342*((abs(u)*1E6)^0.1267))*1E3/rapportIE
  Sum : Sum  Inputs=|++
  Sum1 : Sum  Inputs=|++
  Transfer Fcn : TransferFcn  Numerator=[Rcan]  Denominator=[Rcan*Cmem 1]
  OutZmem : Outport  Orientation=left
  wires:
  Gain/1 -> Transfer Fcn/1
  Transfer Fcn/1 -> Sum/1
  Sum/1 -> Divide/2
  Rext/1 -> Divide1/2
  Constant1/1 -> Divide/1
  Constant/1 -> Divide1/1
  Divide/1 -> Sum1/1
  Constant2/1 -> Divide2/1
  Sum1/1 -> Divide2/2
  Rint/1 -> Sum/2
  Divide1/1 -> Sum1/2
  Contrôleur/2(temp) -> Rext/1, Rint/1, Gain/1
  Divide2/1 -> Contrôleur/2(calc)
  InZmem/1 -> Contrôleur/1(u)
  Contrôleur/1(y) -> OutZmem/1

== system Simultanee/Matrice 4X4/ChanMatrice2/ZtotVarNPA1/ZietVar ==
  InZiet : Inport  Orientation=left  Port=1  LatchInput=off
  Constant{,1..2,4} (4 alike) : Constant
  Contrôleur : Stateflow chart  Orientation=left
  Divide{1..4} (4 alike) : Product  Inputs=*/  OutScaling=2^-10
  Rct : Fcn  Expr=u*(3147.77*(1/((1E6*abs(u))^0.7199)))*1000
  Sum : Sum  Inputs=|++
  Sum1 : Sum  Inputs=|++
  Zcpa : Subsystem
  Zw : Subsystem
  OutZiet : Outport  Orientation=left
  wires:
  Constant/1 -> Divide1/1
  Constant1/1 -> Divide2/1
  Constant2/1 -> Divide3/1
  Zcpa/1(OutZcpa) -> Divide3/2
  Zw/1(OutZw) -> Divide2/2
  Rct/1 -> Divide1/2
  Divide3/1 -> Sum/1
  Constant4/1 -> Divide4/1
  Divide2/1 -> Sum/2
  Sum/1 -> Sum1/1
  Divide1/1 -> Sum1/2
  Sum1/1 -> Divide4/2
  Contrôleur/2(temp) -> Rct/1, Zw/1(InZw), Zcpa/1(InZcpa)
  InZiet/1 -> Contrôleur/1(u)
  Contrôleur/1(y) -> OutZiet/1
  Divide4/1 -> Contrôleur/2(calc)

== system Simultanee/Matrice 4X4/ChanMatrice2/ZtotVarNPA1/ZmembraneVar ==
  InZmem : Inport  Orientation=left  Port=1  LatchInput=off
  Constant : Constant
  Constant1 : Constant
  Constant2 : Constant
  Contrôleur : Stateflow chart  Orientation=left
  Divide : Product  Inputs=*/  OutScaling=2^-10
  Divide1 : Product  Inputs=*/  OutScaling=2^-10
  Divide2 : Product  Inputs=*/  OutScaling=2^-10
  Gain : Gain  Gain=2
  Rext : Fcn  Expr=u*(1.6342*((abs(u)*1E6)^0.1267))*1E3
  Rint : Fcn  Expr=u*(1.6342*((abs(u)*1E6)^0.1267))*1E3/rapportIE
  Sum : Sum  Inputs=|++
  Sum1 : Sum  Inputs=|++
  Transfer Fcn : TransferFcn  Numerator=[Rcan]  Denominator=[Rcan*Cmem 1]
  OutZmem : Outport  Orientation=left
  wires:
  Gain/1 -> Transfer Fcn/1
  Transfer Fcn/1 -> Sum/1
  Sum/1 -> Divide/2
  Rext/1 -> Divide1/2
  Constant1/1 -> Divide/1
  Constant/1 -> Divide1/1
  Divide/1 -> Sum1/1
  Constant2/1 -> Divide2/1
  Sum1/1 -> Divide2/2
  Rint/1 -> Sum/2
  Divide1/1 -> Sum1/2
  Contrôleur/2(temp) -> Rext/1, Rint/1, Gain/1
  Divide2/1 -> Contrôleur/2(calc)
  InZmem/1 -> Contrôleur/1(u)
  Contrôleur/1(y) -> OutZmem/1

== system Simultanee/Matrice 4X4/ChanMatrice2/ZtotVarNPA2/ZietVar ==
  InZiet : Inport  Orientation=left  Port=1  LatchInput=off
  Constant{,1..2,4} (4 alike) : Constant
  Contrôleur : Stateflow chart  Orientation=left
  Divide{1..4} (4 alike) : Product  Inputs=*/  OutScaling=2^-10
  Rct : Fcn  Expr=u*(3147.77*(1/((1E6*abs(u))^0.7199)))*1000
  Sum : Sum  Inputs=|++
  Sum1 : Sum  Inputs=|++
  Zcpa : Subsystem
  Zw : Subsystem
  OutZiet : Outport  Orientation=left
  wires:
  Constant/1 -> Divide1/1
  Constant1/1 -> Divide2/1
  Constant2/1 -> Divide3/1
  Zcpa/1(OutZcpa) -> Divide3/2
  Zw/1(OutZw) -> Divide2/2
  Rct/1 -> Divide1/2
  Divide3/1 -> Sum/1
  Constant4/1 -> Divide4/1
  Divide2/1 -> Sum/2
  Sum/1 -> Sum1/1
  Divide1/1 -> Sum1/2
  Sum1/1 -> Divide4/2
  Contrôleur/2(temp) -> Rct/1, Zw/1(InZw), Zcpa/1(InZcpa)
  InZiet/1 -> Contrôleur/1(u)
  Contrôleur/1(y) -> OutZiet/1
  Divide4/1 -> Contrôleur/2(calc)

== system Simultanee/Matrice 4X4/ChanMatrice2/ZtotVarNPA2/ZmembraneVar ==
  InZmem : Inport  Orientation=left  Port=1  LatchInput=off
  Constant : Constant
  Constant1 : Constant
  Constant2 : Constant
  Contrôleur : Stateflow chart  Orientation=left
  Divide : Product  Inputs=*/  OutScaling=2^-10
  Divide1 : Product  Inputs=*/  OutScaling=2^-10
  Divide2 : Product  Inputs=*/  OutScaling=2^-10
  Gain : Gain  Gain=2
  Rext : Fcn  Expr=u*(1.6342*((abs(u)*1E6)^0.1267))*1E3
  Rint : Fcn  Expr=u*(1.6342*((abs(u)*1E6)^0.1267))*1E3/rapportIE
  Sum : Sum  Inputs=|++
  Sum1 : Sum  Inputs=|++
  Transfer Fcn : TransferFcn  Numerator=[Rcan]  Denominator=[Rcan*Cmem 1]
  OutZmem : Outport  Orientation=left
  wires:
  Gain/1 -> Transfer Fcn/1
  Transfer Fcn/1 -> Sum/1
  Sum/1 -> Divide/2
  Rext/1 -> Divide1/2
  Constant1/1 -> Divide/1
  Constant/1 -> Divide1/1
  Divide/1 -> Sum1/1
  Constant2/1 -> Divide2/1
  Sum1/1 -> Divide2/2
  Rint/1 -> Sum/2
  Divide1/1 -> Sum1/2
  Contrôleur/2(temp) -> Rext/1, Rint/1, Gain/1
  Divide2/1 -> Contrôleur/2(calc)
  InZmem/1 -> Contrôleur/1(u)
  Contrôleur/1(y) -> OutZmem/1

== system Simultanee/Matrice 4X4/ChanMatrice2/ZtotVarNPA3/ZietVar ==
  InZiet : Inport  Orientation=left  Port=1  LatchInput=off
  Constant{,1..2,4} (4 alike) : Constant
  Contrôleur : Stateflow chart  Orientation=left
  Divide{1..4} (4 alike) : Product  Inputs=*/  OutScaling=2^-10
  Rct : Fcn  Expr=u*(3147.77*(1/((1E6*abs(u))^0.7199)))*1000
  Sum : Sum  Inputs=|++
  Sum1 : Sum  Inputs=|++
  Zcpa : Subsystem
  Zw : Subsystem
  OutZiet : Outport  Orientation=left
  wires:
  Constant/1 -> Divide1/1
  Constant1/1 -> Divide2/1
  Constant2/1 -> Divide3/1
  Zcpa/1(OutZcpa) -> Divide3/2
  Zw/1(OutZw) -> Divide2/2
  Rct/1 -> Divide1/2
  Divide3/1 -> Sum/1
  Constant4/1 -> Divide4/1
  Divide2/1 -> Sum/2
  Sum/1 -> Sum1/1
  Divide1/1 -> Sum1/2
  Sum1/1 -> Divide4/2
  Contrôleur/2(temp) -> Rct/1, Zw/1(InZw), Zcpa/1(InZcpa)
  InZiet/1 -> Contrôleur/1(u)
  Contrôleur/1(y) -> OutZiet/1
  Divide4/1 -> Contrôleur/2(calc)

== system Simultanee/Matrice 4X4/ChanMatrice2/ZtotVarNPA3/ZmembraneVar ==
  InZmem : Inport  Orientation=left  Port=1  LatchInput=off
  Constant : Constant
  Constant1 : Constant
  Constant2 : Constant
  Contrôleur : Stateflow chart  Orientation=left
  Divide : Product  Inputs=*/  OutScaling=2^-10
  Divide1 : Product  Inputs=*/  OutScaling=2^-10
  Divide2 : Product  Inputs=*/  OutScaling=2^-10
  Gain : Gain  Gain=2
  Rext : Fcn  Expr=u*(1.6342*((abs(u)*1E6)^0.1267))*1E3
  Rint : Fcn  Expr=u*(1.6342*((abs(u)*1E6)^0.1267))*1E3/rapportIE
  Sum : Sum  Inputs=|++
  Sum1 : Sum  Inputs=|++
  Transfer Fcn : TransferFcn  Numerator=[Rcan]  Denominator=[Rcan*Cmem 1]
  OutZmem : Outport  Orientation=left
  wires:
  Gain/1 -> Transfer Fcn/1
  Transfer Fcn/1 -> Sum/1
  Sum/1 -> Divide/2
  Rext/1 -> Divide1/2
  Constant1/1 -> Divide/1
  Constant/1 -> Divide1/1
  Divide/1 -> Sum1/1
  Constant2/1 -> Divide2/1
  Sum1/1 -> Divide2/2
  Rint/1 -> Sum/2
  Divide1/1 -> Sum1/2
  Contrôleur/2(temp) -> Rext/1, Rint/1, Gain/1
  Divide2/1 -> Contrôleur/2(calc)
  InZmem/1 -> Contrôleur/1(u)
  Contrôleur/1(y) -> OutZmem/1

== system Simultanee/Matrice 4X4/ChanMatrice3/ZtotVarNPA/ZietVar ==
  InZiet : Inport  Orientation=left  Port=1  LatchInput=off
  Constant{,1..2,4} (4 alike) : Constant
  Contrôleur : Stateflow chart  Orientation=left
  Divide{1..4} (4 alike) : Product  Inputs=*/  OutScaling=2^-10
  Rct : Fcn  Expr=u*(3147.77*(1/((1E6*abs(u))^0.7199)))*1000
  Sum : Sum  Inputs=|++
  Sum1 : Sum  Inputs=|++
  Zcpa : Subsystem
  Zw : Subsystem
  OutZiet : Outport  Orientation=left
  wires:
  Constant/1 -> Divide1/1
  Constant1/1 -> Divide2/1
  Constant2/1 -> Divide3/1
  Zcpa/1(OutZcpa) -> Divide3/2
  Zw/1(OutZw) -> Divide2/2
  Rct/1 -> Divide1/2
  Divide3/1 -> Sum/1
  Constant4/1 -> Divide4/1
  Divide2/1 -> Sum/2
  Sum/1 -> Sum1/1
  Divide1/1 -> Sum1/2
  Sum1/1 -> Divide4/2
  Contrôleur/2(temp) -> Rct/1, Zw/1(InZw), Zcpa/1(InZcpa)
  InZiet/1 -> Contrôleur/1(u)
  Contrôleur/1(y) -> OutZiet/1
  Divide4/1 -> Contrôleur/2(calc)

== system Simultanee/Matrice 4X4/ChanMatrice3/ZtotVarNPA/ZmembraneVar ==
  InZmem : Inport  Orientation=left  Port=1  LatchInput=off
  Constant : Constant
  Constant1 : Constant
  Constant2 : Constant
  Contrôleur : Stateflow chart  Orientation=left
  Divide : Product  Inputs=*/  OutScaling=2^-10
  Divide1 : Product  Inputs=*/  OutScaling=2^-10
  Divide2 : Product  Inputs=*/  OutScaling=2^-10
  Gain : Gain  Gain=2
  Rext : Fcn  Expr=u*(1.6342*((abs(u)*1E6)^0.1267))*1E3
  Rint : Fcn  Expr=u*(1.6342*((abs(u)*1E6)^0.1267))*1E3/rapportIE
  Sum : Sum  Inputs=|++
  Sum1 : Sum  Inputs=|++
  Transfer Fcn : TransferFcn  Numerator=[Rcan]  Denominator=[Rcan*Cmem 1]
  OutZmem : Outport  Orientation=left
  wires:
  Gain/1 -> Transfer Fcn/1
  Transfer Fcn/1 -> Sum/1
  Sum/1 -> Divide/2
  Rext/1 -> Divide1/2
  Constant1/1 -> Divide/1
  Constant/1 -> Divide1/1
  Divide/1 -> Sum1/1
  Constant2/1 -> Divide2/1
  Sum1/1 -> Divide2/2
  Rint/1 -> Sum/2
  Divide1/1 -> Sum1/2
  Contrôleur/2(temp) -> Rext/1, Rint/1, Gain/1
  Divide2/1 -> Contrôleur/2(calc)
  InZmem/1 -> Contrôleur/1(u)
  Contrôleur/1(y) -> OutZmem/1

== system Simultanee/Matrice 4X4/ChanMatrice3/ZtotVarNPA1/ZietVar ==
  InZiet : Inport  Orientation=left  Port=1  LatchInput=off
  Constant{,1..2,4} (4 alike) : Constant
  Contrôleur : Stateflow chart  Orientation=left
  Divide{1..4} (4 alike) : Product  Inputs=*/  OutScaling=2^-10
  Rct : Fcn  Expr=u*(3147.77*(1/((1E6*abs(u))^0.7199)))*1000
  Sum : Sum  Inputs=|++
  Sum1 : Sum  Inputs=|++
  Zcpa : Subsystem
  Zw : Subsystem
  OutZiet : Outport  Orientation=left
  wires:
  Constant/1 -> Divide1/1
  Constant1/1 -> Divide2/1
  Constant2/1 -> Divide3/1
  Zcpa/1(OutZcpa) -> Divide3/2
  Zw/1(OutZw) -> Divide2/2
  Rct/1 -> Divide1/2
  Divide3/1 -> Sum/1
  Constant4/1 -> Divide4/1
  Divide2/1 -> Sum/2
  Sum/1 -> Sum1/1
  Divide1/1 -> Sum1/2
  Sum1/1 -> Divide4/2
  Contrôleur/2(temp) -> Rct/1, Zw/1(InZw), Zcpa/1(InZcpa)
  InZiet/1 -> Contrôleur/1(u)
  Contrôleur/1(y) -> OutZiet/1
  Divide4/1 -> Contrôleur/2(calc)

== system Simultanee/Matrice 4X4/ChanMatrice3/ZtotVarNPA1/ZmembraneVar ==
  InZmem : Inport  Orientation=left  Port=1  LatchInput=off
  Constant : Constant
  Constant1 : Constant
  Constant2 : Constant
  Contrôleur : Stateflow chart  Orientation=left
  Divide : Product  Inputs=*/  OutScaling=2^-10
  Divide1 : Product  Inputs=*/  OutScaling=2^-10
  Divide2 : Product  Inputs=*/  OutScaling=2^-10
  Gain : Gain  Gain=2
  Rext : Fcn  Expr=u*(1.6342*((abs(u)*1E6)^0.1267))*1E3
  Rint : Fcn  Expr=u*(1.6342*((abs(u)*1E6)^0.1267))*1E3/rapportIE
  Sum : Sum  Inputs=|++
  Sum1 : Sum  Inputs=|++
  Transfer Fcn : TransferFcn  Numerator=[Rcan]  Denominator=[Rcan*Cmem 1]
  OutZmem : Outport  Orientation=left
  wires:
  Gain/1 -> Transfer Fcn/1
  Transfer Fcn/1 -> Sum/1
  Sum/1 -> Divide/2
  Rext/1 -> Divide1/2
  Constant1/1 -> Divide/1
  Constant/1 -> Divide1/1
  Divide/1 -> Sum1/1
  Constant2/1 -> Divide2/1
  Sum1/1 -> Divide2/2
  Rint/1 -> Sum/2
  Divide1/1 -> Sum1/2
  Contrôleur/2(temp) -> Rext/1, Rint/1, Gain/1
  Divide2/1 -> Contrôleur/2(calc)
  InZmem/1 -> Contrôleur/1(u)
  Contrôleur/1(y) -> OutZmem/1

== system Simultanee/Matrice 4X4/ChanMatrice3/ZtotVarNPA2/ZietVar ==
  InZiet : Inport  Orientation=left  Port=1  LatchInput=off
  Constant{,1..2,4} (4 alike) : Constant
  Contrôleur : Stateflow chart  Orientation=left
  Divide{1..4} (4 alike) : Product  Inputs=*/  OutScaling=2^-10
  Rct : Fcn  Expr=u*(3147.77*(1/((1E6*abs(u))^0.7199)))*1000
  Sum : Sum  Inputs=|++
  Sum1 : Sum  Inputs=|++
  Zcpa : Subsystem
  Zw : Subsystem
  OutZiet : Outport  Orientation=left
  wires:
  Constant/1 -> Divide1/1
  Constant1/1 -> Divide2/1
  Constant2/1 -> Divide3/1
  Zcpa/1(OutZcpa) -> Divide3/2
  Zw/1(OutZw) -> Divide2/2
  Rct/1 -> Divide1/2
  Divide3/1 -> Sum/1
  Constant4/1 -> Divide4/1
  Divide2/1 -> Sum/2
  Sum/1 -> Sum1/1
  Divide1/1 -> Sum1/2
  Sum1/1 -> Divide4/2
  Contrôleur/2(temp) -> Rct/1, Zw/1(InZw), Zcpa/1(InZcpa)
  InZiet/1 -> Contrôleur/1(u)
  Contrôleur/1(y) -> OutZiet/1
  Divide4/1 -> Contrôleur/2(calc)

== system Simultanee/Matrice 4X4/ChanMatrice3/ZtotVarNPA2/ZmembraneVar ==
  InZmem : Inport  Orientation=left  Port=1  LatchInput=off
  Constant : Constant
  Constant1 : Constant
  Constant2 : Constant
  Contrôleur : Stateflow chart  Orientation=left
  Divide : Product  Inputs=*/  OutScaling=2^-10
  Divide1 : Product  Inputs=*/  OutScaling=2^-10
  Divide2 : Product  Inputs=*/  OutScaling=2^-10
  Gain : Gain  Gain=2
  Rext : Fcn  Expr=u*(1.6342*((abs(u)*1E6)^0.1267))*1E3
  Rint : Fcn  Expr=u*(1.6342*((abs(u)*1E6)^0.1267))*1E3/rapportIE
  Sum : Sum  Inputs=|++
  Sum1 : Sum  Inputs=|++
  Transfer Fcn : TransferFcn  Numerator=[Rcan]  Denominator=[Rcan*Cmem 1]
  OutZmem : Outport  Orientation=left
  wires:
  Gain/1 -> Transfer Fcn/1
  Transfer Fcn/1 -> Sum/1
  Sum/1 -> Divide/2
  Rext/1 -> Divide1/2
  Constant1/1 -> Divide/1
  Constant/1 -> Divide1/1
  Divide/1 -> Sum1/1
  Constant2/1 -> Divide2/1
  Sum1/1 -> Divide2/2
  Rint/1 -> Sum/2
  Divide1/1 -> Sum1/2
  Contrôleur/2(temp) -> Rext/1, Rint/1, Gain/1
  Divide2/1 -> Contrôleur/2(calc)
  InZmem/1 -> Contrôleur/1(u)
  Contrôleur/1(y) -> OutZmem/1
